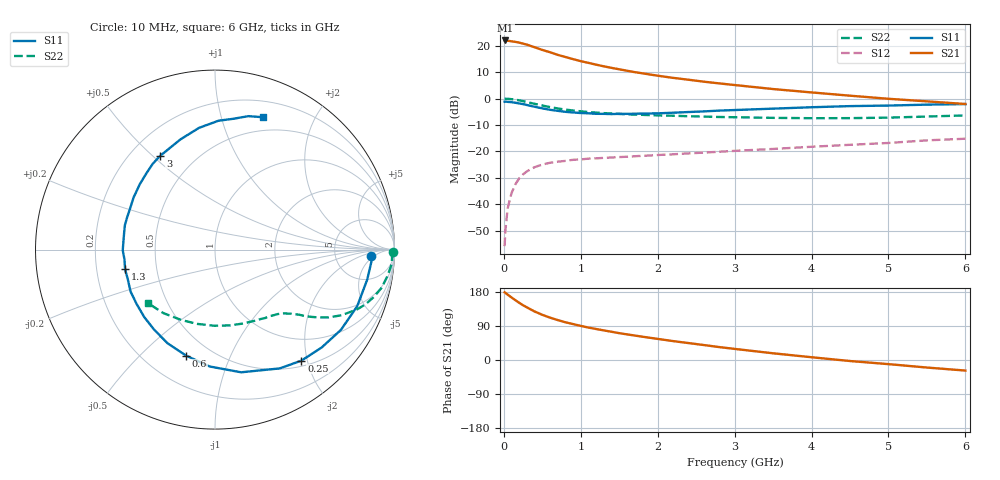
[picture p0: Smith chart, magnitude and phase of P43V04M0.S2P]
! SIEMENS Small Signal Semiconductors
! BFP182
! Si NPN RF Bipolar Junction Transistor in SOT143
! VCE = 3 V  IC = 4 mA
! Common Emitter S-Parameters:  March  1996
# GHz  S  MA  R  50
!  f  S11  S21  S12  S22
! GHz  MAG  ANG  MAG  ANG  MAG  ANG  MAG  ANG
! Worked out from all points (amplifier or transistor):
!   36 points, 10 MHz to 6 GHz, reference 50 ohm
!   highest |S21| = 22.0 dB at 20 MHz (marker M1)
!   |S21| within 3 dB of that: start of sweep to 441.7 MHz
!   unconditionally stable (mu >= 1): 1.742 GHz to 5.526 GHz
!   at 250 MHz: K = 0.18, MSG = 24.8 dB, |S12| = -28.7 dB
!   at 1.4 GHz: K = 0.87, MSG = 17.0 dB, |S12| = -22.3 dB
!   at 6 GHz: K = 0.96, MSG = 6.6 dB, |S12| = -15.2 dB
!   S11 on the Smith chart (normalised r, x): 10 MHz: 13, -4; 250 MHz: 0.59, -1.90; 600 MHz: 0.37, -0.70; 1.3 GHz: 0.33, -0.10; 3 GHz: 0.32, +0.53; 6 GHz: 0.36, +1.37
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0.01  0.8696 -2.2  12.44 178.6  0.0016 86.0  0.9927 -0.9
0.02  0.8738 -4.5  12.58 177.4  0.0032 87.6  0.9872 -1.7
0.05  0.8645 -11.1  12.41 172.4  0.0084 86.6  0.9884 -4.5
0.15  0.8321 -32.5  11.83 157.8  0.0238 71.9  0.9523 -12.9
0.2  0.8067 -42.5  11.45 150.9  0.0308 67.6  0.9235 -16.6
0.25  0.7839 -52.1  10.95 144.4  0.0366 63.0  0.8921 -20.0
0.3  0.7539 -61.4  10.49 138.9  0.0418 58.5  0.8579 -22.9
0.4  0.6989 -78.0  9.352 128.0  0.0501 51.5  0.7943 -27.4
0.5  0.6519 -92.6  8.322 119.2  0.0562 45.7  0.7382 -30.8
0.6  0.6122 -105.3  7.532 111.8  0.0607 41.5  0.6881 -33.3
0.7  0.5849 -116.9  6.717 105.4  0.0636 38.8  0.6493 -35.2
0.8  0.5601 -127.3  6.125 99.6  0.066 36.2  0.6172 -36.7
1  0.5316 -145.2  5.098 90.0  0.0703 32.4  0.573 -38.9
1.1  0.5253 -153.6  4.736 85.6  0.0727 31.6  0.5559 -40.0
1.3  0.5127 -167.8  4.069 78.1  0.0752 30.0  0.5292 -42.2
1.7  0.5152 169.2  3.165 64.6  0.0807 28.8  0.496 -46.8
2.2  0.5385 147.4  2.462 49.9  0.0879 28.3  0.4721 -53.9
3  0.6053 120.2  1.802 29.3  0.102 27.6  0.4423 -68.2
3.5  0.6435 107.4  1.512 17.7  0.111 26.3  0.4306 -78.7
4.5  0.7185 88.4  1.132 -2.7  0.133 23.2  0.4254 -103.2
5.5  0.7663 76.0  0.884 -19.9  0.1614 18.9  0.456 -129.1
6  0.7849 70.0  0.788 -27.9  0.1734 14.8  0.4789 -141.7
